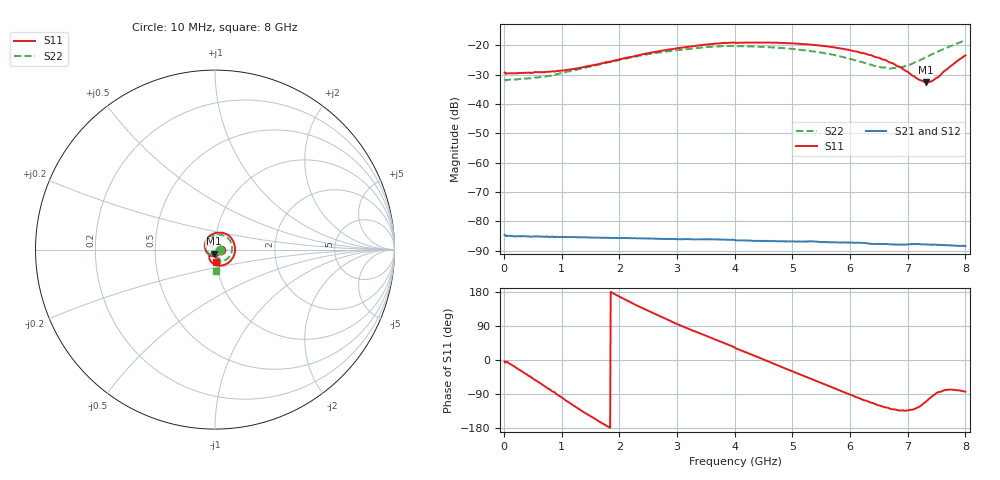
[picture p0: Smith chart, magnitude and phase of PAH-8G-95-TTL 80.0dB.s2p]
! MTS Systemtechnik GmbH
! S-Parameters
! Model: PAH-8G/95-TTL
! Attenuation Step: 80.0dB
! Rohde & Schwarz ZVB8 2Ports - Version 4.11 - 1145.1010k08 SN: 100119
! S2P File Measurements:
! S11 S21 S12 S22
# HZ  S  DB  R  50.00
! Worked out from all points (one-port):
!   800 points, 10 MHz to 8 GHz, reference 50 ohm
!   lowest |S11| = -32.5 dB at 7.31 GHz (marker M1), VSWR 1.05, Z = 49.1 - j2.17 ohm
!   |S11| at or under -10 dB: start of sweep to end of sweep
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1e7  -29.26 -3.7  -84.64 -0.2  -84.37 -0.5  -31.51 -4.3
2.1e8  -29.46 -20.4  -85.10 -29.9  -85.08 -29.9  -31.59 -24.2
7.7e8  -28.94 -75.7  -85.26 -107.5  -85.19 -107.4  -30.45 -87.9
1.35e9  -27.55 -134.7  -85.39 172.4  -85.47 172.3  -27.90 -147.4
2.05e9  -24.52 163.6  -85.66 75.5  -85.67 75.7  -24.71 152.9
2.68e9  -22.00 116.9  -85.91 -11.5  -85.91 -11.1  -22.45 108.0
3.43e9  -19.89 68.5  -86.13 -113.7  -86.15 -114.0  -20.74 59.7
3.79e9  -19.20 46.4  -86.17 -163.5  -86.17 -163.0  -20.24 38.1
4.01e9  -19.13 31.2  -86.43 164.6  -86.50 164.9  -20.27 24.0
4.64e9  -19.04 -7.5  -86.72 78.7  -86.77 78.1  -20.63 -12.5
5.34e9  -19.78 -50.8  -86.78 -18.2  -86.85 -18.0  -21.97 -50.2
5.76e9  -20.80 -76.3  -87.12 -76.9  -87.17 -76.6  -23.41 -69.3
6.11e9  -22.05 -98.0  -87.29 -125.8  -87.26 -126.2  -25.16 -80.8
6.37e9  -23.39 -112.6  -87.65 -162.6  -87.67 -162.9  -26.65 -83.7
6.67e9  -25.64 -126.9  -87.76 156.9  -87.79 157.1  -27.89 -78.4
6.93e9  -28.30 -133.4  -87.91 121.6  -87.95 121.9  -27.26 -69.9
7.18e9  -31.54 -125.1  -87.69 86.5  -87.78 86.8  -25.36 -64.6
7.31e9  -32.53 -110.6  -87.82 67.8  -87.85 67.7  -24.09 -65.0
7.41e9  -32.27 -97.4  -87.86 54.5  -87.92 53.9  -23.20 -66.2
7.52e9  -30.88 -85.4  -88.03 39.0  -87.99 38.6  -22.17 -68.2
7.85e9  -25.40 -79.6  -88.35 -7.0  -88.27 -7.5  -19.38 -79.6
8e9  -23.43 -83.5  -88.41 -27.6  -88.42 -29.0  -18.32 -86.1
